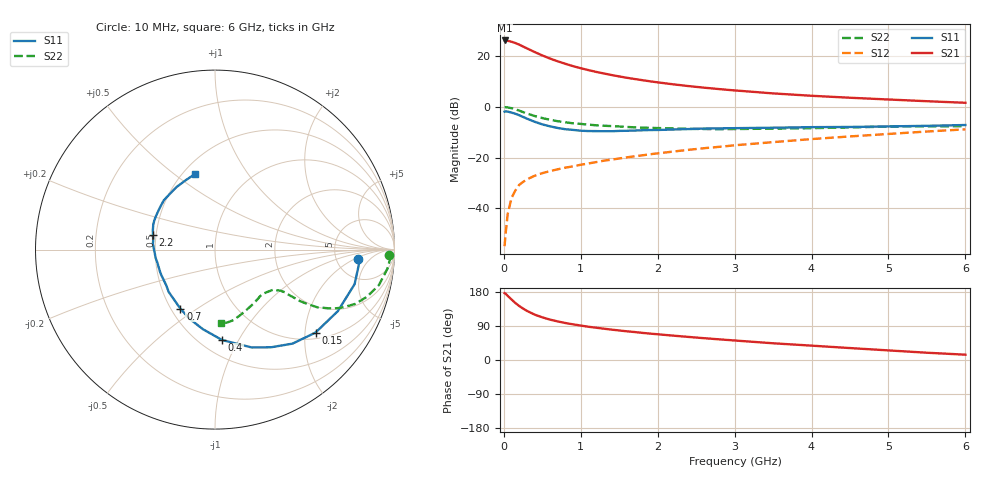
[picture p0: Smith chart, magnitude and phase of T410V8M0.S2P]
! Infineon Technologies  Discrete & RF Semiconductors
! BFR182T
! Si NPN RF Bipolar Junction Transistor in SC75
! VCE = 10 V  IC = 8 mA
! Common Emitter S-Parameters:  October  1999
# GHz  S  MA  R  50
!  f  S11  S21  S12  S22
! GHz  MAG  ANG  MAG  ANG  MAG  ANG  MAG  ANG
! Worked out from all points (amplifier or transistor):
!   36 points, 10 MHz to 6 GHz, reference 50 ohm
!   highest |S21| = 26.1 dB at 10 MHz (marker M1)
!   |S21| within 3 dB of that: start of sweep to 291.9 MHz
!   unconditionally stable (mu >= 1): 1.27 GHz to 4.103 GHz
!   at 250 MHz: K = 0.37, MSG = 26.6 dB, |S12| = -29.6 dB
!   at 1.4 GHz: K = 1.03, MAG = 15.6 dB, |S12| = -20.8 dB
!   at 6 GHz: K = 0.87, MSG = 5.2 dB, |S12| = -8.9 dB
!   S11 on the Smith chart (normalised r, x): 10 MHz: 8.27, -2.36; 150 MHz: 1.16, -2.27; 400 MHz: 0.63, -0.86; 700 MHz: 0.56, -0.43; 2.2 GHz: 0.48, +0.09; 6 GHz: 0.57, +0.60
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0.01  0.799 -3.7  20.11 176.3  0.0018 78.3  0.9721 -1.9
0.02  0.8092 -4.1  19.95 175.5  0.0029 81.6  0.9792 -2.6
0.05  0.8013 -13.9  19.79 169.2  0.0077 86.7  0.9666 -6.3
0.1  0.7655 -26.6  18.96 159.7  0.016 77.2  0.9345 -12.2
0.15  0.7263 -39.5  17.88 150.4  0.0225 71.7  0.8872 -17.2
0.2  0.6789 -50.5  16.62 142.5  0.029 67.7  0.8373 -21.2
0.25  0.6281 -60.0  15.29 135.7  0.0331 63.2  0.784 -24.2
0.3  0.5825 -69.4  14.04 129.6  0.0371 62.1  0.7375 -26.5
0.4  0.5059 -85.4  11.91 119.8  0.0437 58.5  0.6558 -29.4
0.5  0.449 -98.5  10.21 112.6  0.0492 57.2  0.5978 -30.5
0.6  0.4105 -110.4  8.851 106.6  0.054 56.7  0.5527 -31.2
0.7  0.3814 -120.4  7.817 101.8  0.0586 57.0  0.5179 -31.3
0.9  0.3495 -137.6  6.276 94.1  0.0671 58.4  0.4712 -31.5
1.1  0.3315 -151.6  5.247 87.7  0.0763 59.7  0.4432 -31.8
1.4  0.3289 -167.3  4.198 80.2  0.0907 61.2  0.4155 -33.2
1.6  0.3359 -176.1  3.706 75.7  0.1009 61.9  0.3992 -34.1
2.2  0.3552 166.7  2.758 64.3  0.1308 63.0  0.3735 -39.4
2.8  0.3748 154.6  2.219 54.5  0.1622 62.5  0.3608 -46.1
3.5  0.3856 143.1  1.826 44.1  0.2008 60.9  0.3699 -54.8
4.5  0.3992 129.5  1.5 31.5  0.2599 57.4  0.3907 -68.6
5.5  0.4201 112.6  1.282 19.2  0.3247 52.6  0.4118 -80.4
6  0.4362 104.5  1.193 14.0  0.3584 49.3  0.4123 -85.2
